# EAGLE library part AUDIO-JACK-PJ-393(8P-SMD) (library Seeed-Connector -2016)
320040009
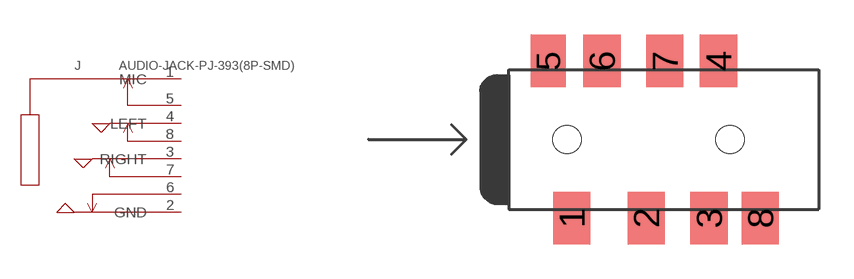
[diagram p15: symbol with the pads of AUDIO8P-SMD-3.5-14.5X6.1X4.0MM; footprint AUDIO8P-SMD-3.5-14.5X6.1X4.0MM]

Designator prefix J

## AUDIO-JACK-PJ-393(8P-SMD) (MPN: PJ-393; VALUE: PJ-393)  [AUDIO8P-SMD-3.5-14.5X6.1X4.0MM]
1  MIC
2  GND
3  RIGHT
4  LEFT
5  5
6  6
7  7
8  8

## Footprint AUDIO8P-SMD-3.5-14.5X6.1X4.0MM (pad centres in mm)
smd 1.6 x 2.25: 1 3.9,-3.375; 2 7.1,-3.375; 3 9.8,-3.375; 4 10.2,3.375; 6 5.2,3.375; 7 7.9,3.375; 8 12,-3.375
smd 1.5 x 2.25: 5 2.9,3.375
hole 1.2 at 3.7,0
hole 1.2 at 10.7,0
